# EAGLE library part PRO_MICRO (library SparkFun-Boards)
SparkFun Pro Micro Atmega32U4 compatible footprint. SparkFun Products: 3.3V/8MHz 5V/16MHz
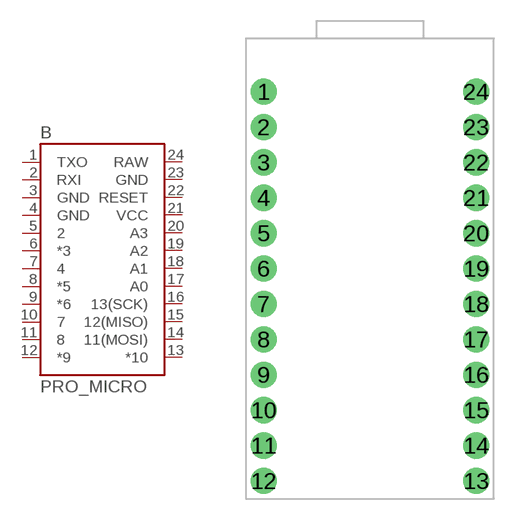
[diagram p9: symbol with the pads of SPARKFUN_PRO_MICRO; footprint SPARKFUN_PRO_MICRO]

Designator prefix B

## PRO_MICRO  [SPARKFUN_PRO_MICRO]
1  TXO
2  RXI
3  GND
4  GND
5  2
6  *3
7  4
8  *5
9  *6
10  7
11  8
12  *9
13  *10
14  11(MOSI)
15  12(MISO)
16  13(SCK)
17  A0
18  A1
19  A2
20  A3
21  VCC
22  RESET
23  GND
24  RAW

## Footprint SPARKFUN_PRO_MICRO (pad centres in mm)
drill 1.016 pad 1.88: 1 -7.62,12.7; 2 -7.62,10.16; 3 -7.62,7.62; 4 -7.62,5.08; 5 -7.62,2.54; 6 -7.62,0; 7 -7.62,-2.54; 8 -7.62,-5.08; 9 -7.62,-7.62; 10 -7.62,-10.16; 11 -7.62,-12.7; 12 -7.62,-15.24; 13 7.62,-15.24; 14 7.62,-12.7; 15 7.62,-10.16; 16 7.62,-7.62; 17 7.62,-5.08; 18 7.62,-2.54; 19 7.62,0; 20 7.62,2.54; 21 7.62,5.08; 22 7.62,7.62; 23 7.62,10.16; 24 7.62,12.7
